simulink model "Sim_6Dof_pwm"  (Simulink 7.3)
settings: Solver=ode4  StartTime=0.0  StopTime=80  FixedStep=0.0005  MaxStep=0.0005  RelTol=1e-3
StopFcn:
  | Pl
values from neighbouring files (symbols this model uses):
  calfa = cos(alfa0*d2r)    [run.m]
  d2r = pi/180    (= 0.0174532925199)    [run.m]
  klr = [0.82083770557  -0.70145835124   0.75722294555   0.32691190448   0.14993771995;        0.55253708187   0.66141640307  -0.4963339086    0.20601876795  -0.07844376733]    [run.m]
  kls = [0.23009875115  -1.3857134134    0.5565800989    0.03843893525  0.1360972015;        0.22658853965   0.3268097242   -0.0904376422    0.0272194403  -0.00768778705]    [run.m]
  r2d = 180/pi    (= 57.2957795131)    [Pl.m]    (also in run.m)
  salfa = sin(alfa0*d2r)    [run.m]
  Thet0 = 43    [run.m]
  V0 = 18640    [run.m]
undefined symbols (not defined in the file or in its folder): A6d, B6d, C6d, D6d, KSmix, Pos_Thrust3

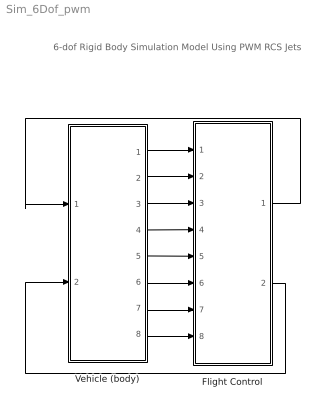
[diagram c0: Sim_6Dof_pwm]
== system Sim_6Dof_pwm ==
  note: 6-dof Rigid Body Simulation Model Using PWM RCS Jets
  Flight Control : Subsystem
  Vehicle (body) : Subsystem
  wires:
  Vehicle (body)/2(p) -> Flight Control/2(pb)
  Vehicle (body)/3(r) -> Flight Control/3(rb)
  Vehicle (body)/6(q) -> Flight Control/6(q)
  Vehicle (body)/5(thet) -> Flight Control/5(thet)
  Vehicle (body)/7(alf) -> Flight Control/7(alfa)
  Vehicle (body)/4(bet) -> Flight Control/4(beta)
  Vehicle (body)/1(phi) -> Flight Control/1(phi)
  Flight Control/2(Aer_pqr) -> Vehicle (body)/2(Aer_pqr)
  Vehicle (body)/8(Nz) -> Flight Control/8(Nz)
  Flight Control/1(Jet_pqr) -> Vehicle (body)/1(Jet_pqr_Nz)

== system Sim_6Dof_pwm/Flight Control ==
  note: Flight Control System
  phi : Inport  OutDataType=sfix(16)  OutScaling=2^0
  pb : Inport  Port=2  OutDataType=sfix(16)  OutScaling=2^0
  rb : Inport  Port=3  OutDataType=sfix(16)  OutScaling=2^0
  beta : Inport  Port=4  OutDataType=sfix(16)  OutScaling=2^0
  thet : Inport  Port=5  OutDataType=sfix(16)  OutScaling=2^0
  q : Inport  Port=6  OutDataType=sfix(16)  OutScaling=2^0
  alfa : Inport  Port=7  OutDataType=sfix(16)  OutScaling=2^0
  Nz : Inport  Port=8  OutDataType=sfix(16)  OutScaling=2^0
  2 deg  Alfa-Comd : Constant  Value=1*d2r  OutDataType=sfix(16)  OutScaling=2^0
  30 deg  phi-cmd : Constant  Value=40*d2r  OutDataType=sfix(16)  OutScaling=2^0
  Body 2 Stabil : Subsystem
  Lateral  Flight Control : Subsystem
  Mix : Subsystem
  Mux1 : Mux  Inputs=[3,1]
  Pitch Flight Control : Subsystem
  Jet_pqr : Outport  OutDataType=sfix(16)  OutScaling=2^0
  Aer_pqr : Outport  Port=2  OutDataType=sfix(16)  OutScaling=2^0
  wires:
  Lateral  Flight Control/1(rcs_PR) -> Mix/1(Rcs_PR)
  Lateral  Flight Control/2(aero_PR) -> Mix/2(Aer_PR)
  Pitch Flight Control/1(rcs_Q) -> Mix/3(Rcs_Q)
  Pitch Flight Control/2(aero_Q) -> Mix/4(Aer_Q)
  beta/1 -> Lateral  Flight Control/3(beta)
  Mix/2(Aer_pqr) -> Aer_pqr/1  "3"
  thet/1 -> Pitch Flight Control/1(thet)
  q/1 -> Pitch Flight Control/2(q)
  alfa/1 -> Pitch Flight Control/3(alf)
  Body 2 Stabil/2(r_s) -> Lateral  Flight Control/2(rs)
  Body 2 Stabil/1(p_s) -> Lateral  Flight Control/1(ps)
  rb/1 -> Body 2 Stabil/3(r_b)
  pb/1 -> Body 2 Stabil/2(p_b)
  phi/1 -> Body 2 Stabil/1(phi)
  Nz/1 -> Pitch Flight Control/4(Nz)
  Mix/1(Jet_pqr) -> Mux1/1  "3"
  2 deg  Alfa-Comd/1 -> Pitch Flight Control/5(alf-cmd)
  30 deg  phi-cmd/1 -> Lateral  Flight Control/4(phi-cmd)
  Pitch Flight Control/3(Nzfb) -> Mux1/2
  Mux1/1 -> Jet_pqr/1

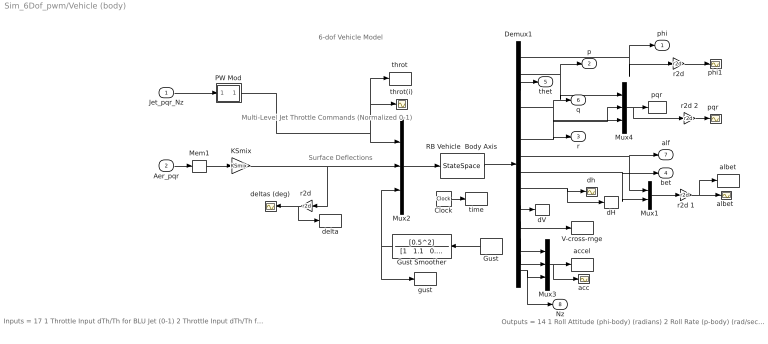
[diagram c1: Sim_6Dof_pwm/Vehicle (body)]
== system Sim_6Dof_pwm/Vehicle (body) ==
  note: Surface Deflections
  note: Multi-Level Jet Throttle Commands (Normalized 0-1)
  note: 6-dof Vehicle Model
  note: Inputs = 17 1 Throttle Input dTh/Th for BLU Jet (0-1) 2 Throttle Input dTh/Th for BRU Jet (0-1) 3 Throttle Input dTh/Th for BLD Jet (0-1) 4 Throttle Input dTh/Th for BRD Jet (0-1) 5 Throttle Input dTh/Th for BL+Y Jet (0-1) 6 Throttle Input dTh/Th for BR-Y Jet (0-1) 7 Throttle Input dTh/Th for FU Jet (0-1) 8 Throttle Input dTh/Th for FLD Jet (0-1) 9 Throttle Input dTh/Th for FRD Jet (0-1) 10 Throttle Input dTh/Th for FL+Y Jet (0-1) 11 Throttle Input dTh/Th for FR-Y Jet (0-1) 12 Left Outbrd Elevon Deflection (radians) 13 Left Inboard Elevon Deflection (radians) 14 Right Inbrd Elevon Deflection (radians) 15 Right Outbrd Elevon Deflection (radians) 16 Vertical Rudder Deflection (radians) 17 Gust Veloc, Azim-Elev Angles=(45,90) (deg)
  note: Outputs = 14 1 Roll Attitude (phi-body) (radians) 2 Roll Rate (p-body) (rad/sec) 3 Pitch Attitude (thet-bdy) (radians) 4 Pitch Rate (q-body) (rad/sec) 5 Yaw Attitude (psi-body) (radians) 6 Yaw Rate (r-body) (rad/sec) 7 Angle of attack, alfa, (radians) 8 Angle of sideslip, beta, (radian) 9 Change in Altitude, delta-h, (feet) 10 Forward Acceleration (V-dot) (ft/sec) 11 Cross Range Velocity (Vcr) (ft/sec) 12 CG Acceleration along X axis, (ft/sec^2) 13 CG Acceleration along Y axis, (ft/sec^2) 14 CG Acceleration along Z axis, (ft/sec^2)
  Jet_pqr_Nz : Inport  OutDataType=sfix(16)  OutScaling=2^0
  Aer_pqr : Inport  Port=2  OutDataType=sfix(16)  OutScaling=2^0
  Clock : Clock
  Demux1 : Demux  Outputs=14
  Gust : DiscretePulseGenerator  PulseType=Time based  Amplitude=50  Period=500  PulseWidth=10  PhaseDelay=0  SampleTime=1
  Gust Smoother : TransferFcn  Numerator=[0.5^2]  Denominator="[1   1.1   0.5^2]"
  KSmix : Gain  Gain=KSmix  Multiplication=Matrix(K*u)  ParameterDataType=sfix(16)  ParameterScaling=2^0  OutDataType=sfix(16)  OutScaling=2^0
  Mem1 : Memory
  Mux1 : Mux  Inputs=2
  Mux2 : Mux  Inputs=[11, 5, 1]
  Mux3 : Mux  Inputs=3
  Mux4 : Mux  Inputs=3
  PW Mod : Subsystem
  RB Vehicle  Body Axis : StateSpace  A=A6d  B=B6d  C=C6d  D=D6d
  V-cross-rnge : ToWorkspace  VariableName=Vxrng  SampleTime=-1  SaveFormat=Array
  acc : Scope
  accel : ToWorkspace  VariableName=accel  SampleTime=-1  SaveFormat=Array
  albet : ToWorkspace  VariableName=albet  SampleTime=-1  SaveFormat=Array
  "albet " : Scope
  dH : ToWorkspace  VariableName=dH  SampleTime=-1  SaveFormat=Array
  dV : ToWorkspace  VariableName=dV  SampleTime=-1  SaveFormat=Array
  delta : ToWorkspace  VariableName=delta  SampleTime=-1  SaveFormat=Array
  deltas (deg) : Scope
  dh : Scope
  gust : ToWorkspace  VariableName=gust  SampleTime=-1  SaveFormat=Array
  phi1 : Scope
  pqr : ToWorkspace  VariableName=pqr  SampleTime=-1  SaveFormat=Array
  "pqr  " : Scope
  r2d : Gain  Gain=r2d  ParameterDataType=sfix(16)  ParameterScaling=2^0  OutDataType=sfix(16)  OutScaling=2^0
  "r2d " : Gain  Gain=r2d  ParameterDataType=sfix(16)  ParameterScaling=2^0  OutDataType=sfix(16)  OutScaling=2^0
  r2d 1 : Gain  Gain=r2d  ParameterDataType=sfix(16)  ParameterScaling=2^0  OutDataType=sfix(16)  OutScaling=2^0
  r2d 2 : Gain  Gain=r2d  ParameterDataType=sfix(16)  ParameterScaling=2^0  OutDataType=sfix(16)  OutScaling=2^0
  throt : ToWorkspace  VariableName=throt  SampleTime=-1  SaveFormat=Array
  throt(i) : Scope
  time : ToWorkspace  VariableName=time  SampleTime=-1  SaveFormat=Array
  phi : Outport  OutDataType=sfix(16)  OutScaling=2^0
  p : Outport  Port=2  OutDataType=sfix(16)  OutScaling=2^0
  r : Outport  Port=3  OutDataType=sfix(16)  OutScaling=2^0
  bet : Outport  Port=4  OutDataType=sfix(16)  OutScaling=2^0
  thet : Outport  Port=5  OutDataType=sfix(16)  OutScaling=2^0
  q : Outport  Port=6  OutDataType=sfix(16)  OutScaling=2^0
  alf : Outport  Port=7  OutDataType=sfix(16)  OutScaling=2^0
  Nz : Outport  Port=8  OutDataType=sfix(16)  OutScaling=2^0
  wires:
  Mux2/1 -> RB Vehicle  Body Axis/1
  KSmix/1 -> Mux2/2, "r2d "/1
  Demux1/2 -> p/1, Mux4/1
  Demux1/4 -> q/1, Mux4/2
  Demux1/6 -> r/1, Mux4/3
  Demux1/7 -> alf/1, Mux1/1
  Demux1/8 -> bet/1, Mux1/2
  Aer_pqr/1 -> Mem1/1
  Demux1/3 -> thet/1
  "r2d "/1 -> deltas (deg)/1, delta/1
  Demux1/1 -> phi/1, r2d/1
  RB Vehicle  Body Axis/1 -> Demux1/1
  Demux1/9 -> dh/1, dH/1
  Demux1/10 -> dV/1
  r2d 1/1 -> "albet "/1, albet/1
  Demux1/11 -> V-cross-rnge/1
  Gust Smoother/1 -> gust/1, Mux2/3
  r2d/1 -> phi1/1
  Jet_pqr_Nz/1 -> PW Mod/1(In)
  Mem1/1 -> KSmix/1
  Clock/1 -> time/1
  Mux1/1 -> r2d 1/1
  Demux1/14 -> Mux3/3, Nz/1
  Demux1/13 -> Mux3/2
  Demux1/12 -> Mux3/1
  Mux3/1 -> accel/1, acc/1
  Mux4/1 -> pqr/1, r2d 2/1
  r2d 2/1 -> "pqr  "/1
  Gust/1 -> Gust Smoother/1
  PW Mod/1(Ot) -> Mux2/1, throt(i)/1, throt/1

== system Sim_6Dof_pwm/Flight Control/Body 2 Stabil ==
  note: Body to Stability Axes Transformation
  phi : Inport  OutDataType=sfix(16)  OutScaling=2^0
  p_b : Inport  Port=2  OutDataType=sfix(16)  OutScaling=2^0
  r_b : Inport  Port=3  OutDataType=sfix(16)  OutScaling=2^0
  Mux1 : Mux  Inputs=2
  Sum1 : Sum  Inputs=+|+  OutDataType=sfix(16)  OutScaling=2^0
  Sum2 : Sum  Inputs=+|-  OutDataType=sfix(16)  OutScaling=2^0
  Sum3 : Sum  Inputs=|++  OutDataType=sfix(16)  OutScaling=2^0
  Sum4 : Sum  Inputs=|+-  OutDataType=sfix(16)  OutScaling=2^0
  calfa : Gain  Gain=calfa  ParameterDataType=sfix(16)  ParameterScaling=2^0  OutDataType=sfix(16)  OutScaling=2^0
  "calfa " : Gain  Gain=calfa  ParameterDataType=sfix(16)  ParameterScaling=2^0  OutDataType=sfix(16)  OutScaling=2^0
  g cos(Thet0) /V0 : Gain  Gain=32.2*cos(Thet0*d2r)/V0  ParameterDataType=sfix(16)  ParameterScaling=2^0  OutDataType=sfix(16)  OutScaling=2^0
  g sin(Thet0) /V0 : Gain  Gain=32.2*sin(Thet0*d2r)/V0  ParameterDataType=sfix(16)  ParameterScaling=2^0  OutDataType=sfix(16)  OutScaling=2^0
  pr_stabil : ToWorkspace  VariableName=pr_st  SampleTime=-1  SaveFormat=Array
  salfa : Gain  Gain=salfa  ParameterDataType=sfix(16)  ParameterScaling=2^0  OutDataType=sfix(16)  OutScaling=2^0
  "salfa " : Gain  Gain=salfa  ParameterDataType=sfix(16)  ParameterScaling=2^0  OutDataType=sfix(16)  OutScaling=2^0
  p_s : Outport  OutDataType=sfix(16)  OutScaling=2^0
  r_s : Outport  Port=2  OutDataType=sfix(16)  OutScaling=2^0
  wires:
  Sum1/1 -> p_s/1, Mux1/1
  Sum2/1 -> r_s/1, Mux1/2
  p_b/1 -> Sum3/1
  r_b/1 -> Sum4/1
  g cos(Thet0) /V0/1 -> Sum3/2
  g sin(Thet0) /V0/1 -> Sum4/2
  phi/1 -> g cos(Thet0) /V0/1, g sin(Thet0) /V0/1
  Sum4/1 -> "calfa "/1, salfa/1
  Sum3/1 -> "salfa "/1, calfa/1
  calfa/1 -> Sum1/1
  salfa/1 -> Sum1/2
  "calfa "/1 -> Sum2/1
  "salfa "/1 -> Sum2/2
  Mux1/1 -> pr_stabil/1

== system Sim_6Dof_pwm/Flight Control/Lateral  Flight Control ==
  note: Lateral Flight Control System
  ps : Inport  OutDataType=sfix(16)  OutScaling=2^0
  rs : Inport  Port=2  OutDataType=sfix(16)  OutScaling=2^0
  beta : Inport  Port=3  OutDataType=sfix(16)  OutScaling=2^0
  phi-cmd : Inport  Port=4  OutDataType=sfix(16)  OutScaling=2^0
  5 state Aero feedback : Gain  Gain=-kls  Multiplication=Matrix(K*u)  ParameterDataType=sfix(16)  ParameterScaling=2^0  OutDataType=sfix(16)  OutScaling=2^0
  5 state RCS feedback : Gain  Gain=-klr  Multiplication=Matrix(K*u)  ParameterDataType=sfix(16)  ParameterScaling=2^0  OutDataType=sfix(16)  OutScaling=2^0
  Int : Integrator
  "Int " : Integrator
  Mux3 : Mux  Inputs=5
  Sum : Sum  Inputs=|+-  OutDataType=sfix(16)  OutScaling=2^0
  phi : Scope
  phi-cmd (rad) : ToWorkspace  VariableName=phi_cmd  SampleTime=-1  SaveFormat=Array
  phi-stabil : ToWorkspace  VariableName=phi_st  SampleTime=-1  SaveFormat=Array
  r2d : Gain  Gain=r2d  ParameterDataType=sfix(16)  ParameterScaling=2^0  OutDataType=sfix(16)  OutScaling=2^0
  rcs_PR : Outport  OutDataType=sfix(16)  OutScaling=2^0
  aero_PR : Outport  Port=2  OutDataType=sfix(16)  OutScaling=2^0
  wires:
  "Int "/1 -> Sum/1, r2d/1  "pint"
  Sum/1 -> Mux3/4
  Int/1 -> Mux3/5  "beti"
  beta/1 -> Int/1, Mux3/3
  ps/1 -> "Int "/1, Mux3/1
  Mux3/1 -> 5 state Aero feedback/1, 5 state RCS feedback/1
  rs/1 -> Mux3/2
  5 state RCS feedback/1 -> rcs_PR/1  "rcs(P,R)"
  5 state Aero feedback/1 -> aero_PR/1  "aero(P,R)"
  phi-cmd/1 -> Sum/2, phi-cmd (rad)/1
  r2d/1 -> phi/1, phi-stabil/1

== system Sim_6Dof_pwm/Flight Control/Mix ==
  Rcs_PR : Inport  OutDataType=sfix(16)  OutScaling=2^0
  Aer_PR : Inport  Port=2  OutDataType=sfix(16)  OutScaling=2^0
  Rcs_Q : Inport  Port=3  OutDataType=sfix(16)  OutScaling=2^0
  Aer_Q : Inport  Port=4  OutDataType=sfix(16)  OutScaling=2^0
  Demux1 : Demux  Outputs=2
  Demux2 : Demux  Outputs=2
  Mux1 : Mux  Inputs=3
  Mux2 : Mux  Inputs=3
  Jet_pqr : Outport  OutDataType=sfix(16)  OutScaling=2^0
  Aer_pqr : Outport  Port=2  OutDataType=sfix(16)  OutScaling=2^0
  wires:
  Demux1/1 -> Mux1/1
  Demux1/2 -> Mux1/3
  Demux2/1 -> Mux2/1
  Demux2/2 -> Mux2/3
  Mux1/1 -> Jet_pqr/1
  Rcs_PR/1 -> Demux1/1
  Aer_PR/1 -> Demux2/1
  Aer_Q/1 -> Mux2/2
  Mux2/1 -> Aer_pqr/1
  Rcs_Q/1 -> Mux1/2

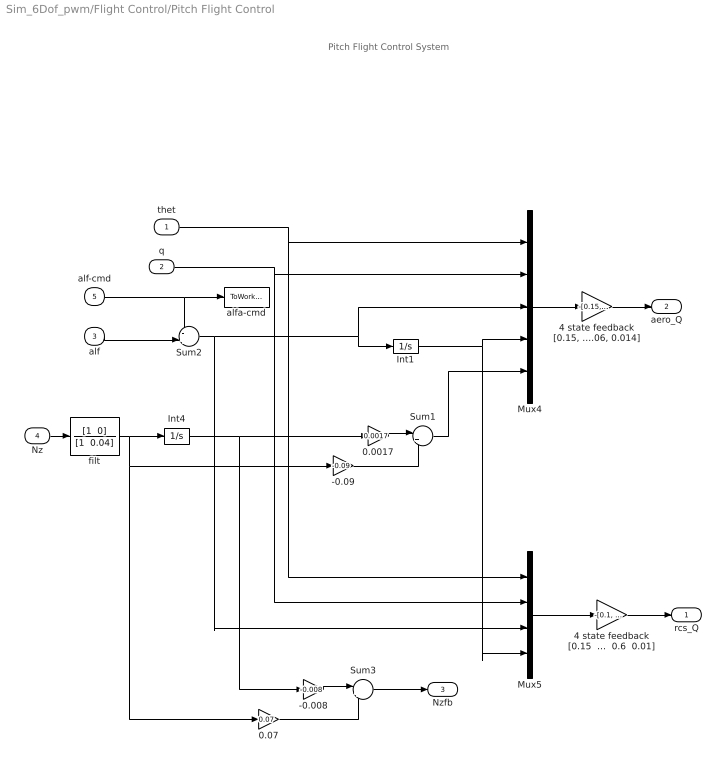
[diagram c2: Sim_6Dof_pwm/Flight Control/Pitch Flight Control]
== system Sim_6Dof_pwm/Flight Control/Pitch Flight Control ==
  note: Pitch Flight Control System
  thet : Inport  OutDataType=sfix(16)  OutScaling=2^0
  q : Inport  Port=2  OutDataType=sfix(16)  OutScaling=2^0
  alf : Inport  Port=3  OutDataType=sfix(16)  OutScaling=2^0
  Nz : Inport  Port=4  OutDataType=sfix(16)  OutScaling=2^0
  alf-cmd : Inport  Port=5  OutDataType=sfix(16)  OutScaling=2^0
  -0.008 : Gain  Gain=-0.008  ParameterDataType=sfix(16)  ParameterScaling=2^0  OutDataType=sfix(16)  OutScaling=2^0
  -0.09 : Gain  Gain=-0.09  ParameterDataType=sfix(16)  ParameterScaling=2^0  OutDataType=sfix(16)  OutScaling=2^0
  0.0017 : Gain  Gain=0.0017  ParameterDataType=sfix(16)  ParameterScaling=2^0  OutDataType=sfix(16)  OutScaling=2^0
  0.07 : Gain  Gain=0.07  ParameterDataType=sfix(16)  ParameterScaling=2^0  OutDataType=sfix(16)  OutScaling=2^0
  4 state feedback [0.15  1.8  0.6  0.01] : Gain  Gain="-[0.1,   1.8,   0.9,    0.01]"  Multiplication=Matrix(K*u)  ParameterDataType=sfix(16)  ParameterScaling=2^0  OutDataType=sfix(16)  OutScaling=2^0
  "4 state feedback [0.15, 2, 0.9, 0.06, 0.014]" : Gain  Gain="-[0.15,   2,   1.2,    0.09,   0.015]"  Multiplication=Matrix(K*u)  ParameterDataType=sfix(16)  ParameterScaling=2^0  OutDataType=sfix(16)  OutScaling=2^0
  Int1 : Integrator
  Int4 : Integrator
  Mux4 : Mux  Inputs=5
  Mux5 : Mux
  Sum1 : Sum  Inputs=|++  OutDataType=sfix(16)  OutScaling=2^0
  Sum2 : Sum  Inputs=-+|  OutDataType=sfix(16)  OutScaling=2^0
  Sum3 : Sum  Inputs=|++  OutDataType=sfix(16)  OutScaling=2^0
  alfa-cmd : ToWorkspace  VariableName=alfa_cmd  SampleTime=-1  SaveFormat=Array
  filt : TransferFcn  Numerator="[1  0]"  Denominator="[1  0.04]"
  rcs_Q : Outport  OutDataType=sfix(16)  OutScaling=2^0
  aero_Q : Outport  Port=2  OutDataType=sfix(16)  OutScaling=2^0
  Nzfb : Outport  Port=3  OutDataType=sfix(16)  OutScaling=2^0
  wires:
  alf-cmd/1 -> Sum2/1, alfa-cmd/1
  alf/1 -> Sum2/2
  filt/1 -> 0.07/1, -0.09/1, Int4/1
  Int4/1 -> -0.008/1, 0.0017/1
  -0.008/1 -> Sum3/1
  0.07/1 -> Sum3/2
  4 state feedback [0.15  1.8  0.6  0.01]/1 -> rcs_Q/1
  Mux5/1 -> 4 state feedback [0.15  1.8  0.6  0.01]/1
  "4 state feedback [0.15, 2, 0.9, 0.06, 0.014]"/1 -> aero_Q/1
  Mux4/1 -> "4 state feedback [0.15, 2, 0.9, 0.06, 0.014]"/1
  Sum1/1 -> Mux4/5
  Nz/1 -> filt/1
  -0.09/1 -> Sum1/2
  0.0017/1 -> Sum1/1
  q/1 -> Mux5/2, Mux4/2
  thet/1 -> Mux5/1, Mux4/1
  Sum2/1 -> Mux5/3, Mux4/3, Int1/1
  Int1/1 -> Mux5/4, Mux4/4
  Sum3/1 -> Nzfb/1

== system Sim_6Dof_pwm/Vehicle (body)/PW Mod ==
  note: Jet Selection Logic
  In : Inport  OutDataType=sfix(16)  OutScaling=2^0
  Demux2 : Demux  Outputs="[3  3  3  3  3  3  2  2  2  2  2  1]"
  Mem : Memory
  Mix Logic +ve thrusts : MATLABFcn  MATLABFcn=Pos_Thrust3(u(1:4) )  OutputDimensions=6*3 + 5*2 + 1  OutputSignalType=real
  Mux1 : Mux  Inputs=11
  PW Modulators : Subsystem
  error : Scope
  error-magn : ToWorkspace  VariableName=erm  SampleTime=-1  SaveFormat=Array
  Ot : Outport  OutDataType=sfix(16)  OutScaling=2^0
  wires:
  In/1 -> Mem/1
  Mux1/1 -> Ot/1
  Mem/1 -> Mix Logic +ve thrusts/1
  Demux2/1 -> PW Modulators/1(In)
  Demux2/2 -> PW Modulators/2(In1)
  Demux2/3 -> PW Modulators/3(In2)
  Demux2/4 -> PW Modulators/4(In3)
  Demux2/5 -> PW Modulators/5(In4)
  Demux2/6 -> PW Modulators/6(In5)
  Demux2/7 -> PW Modulators/7(In6)
  Demux2/8 -> PW Modulators/8(In7)
  Demux2/9 -> PW Modulators/9(In8)
  Demux2/10 -> PW Modulators/10(In9)
  Demux2/11 -> PW Modulators/11(In10)
  PW Modulators/1(O) -> Mux1/1
  PW Modulators/2(O1) -> Mux1/2
  PW Modulators/3(O2) -> Mux1/3
  PW Modulators/4(O3) -> Mux1/4
  PW Modulators/5(O4) -> Mux1/5
  PW Modulators/6(O5) -> Mux1/6
  PW Modulators/7(O6) -> Mux1/7
  PW Modulators/8(O7) -> Mux1/8
  PW Modulators/9(O8) -> Mux1/9
  PW Modulators/10(O9) -> Mux1/10
  PW Modulators/11(O10) -> Mux1/11
  Mix Logic +ve thrusts/1 -> Demux2/1
  Demux2/12 -> error/1, error-magn/1

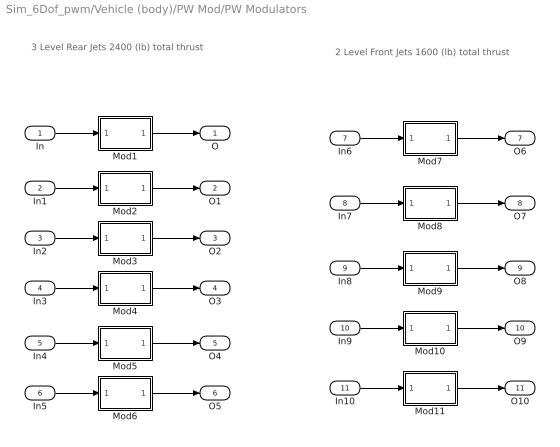
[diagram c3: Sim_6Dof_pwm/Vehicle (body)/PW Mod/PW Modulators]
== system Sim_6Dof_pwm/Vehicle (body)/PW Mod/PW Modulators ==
  note: 3 Level Rear Jets 2400 (lb) total thrust
  note: 2 Level Front Jets 1600 (lb) total thrust
  In : Inport  OutDataType=sfix(16)  OutScaling=2^0
  In1 : Inport  Port=2  OutDataType=sfix(16)  OutScaling=2^0
  In2 : Inport  Port=3  OutDataType=sfix(16)  OutScaling=2^0
  In3 : Inport  Port=4  OutDataType=sfix(16)  OutScaling=2^0
  In4 : Inport  Port=5  OutDataType=sfix(16)  OutScaling=2^0
  In5 : Inport  Port=6  OutDataType=sfix(16)  OutScaling=2^0
  In6 : Inport  Port=7  OutDataType=sfix(16)  OutScaling=2^0
  In7 : Inport  Port=8  OutDataType=sfix(16)  OutScaling=2^0
  In8 : Inport  Port=9  OutDataType=sfix(16)  OutScaling=2^0
  In9 : Inport  Port=10  OutDataType=sfix(16)  OutScaling=2^0
  In10 : Inport  Port=11  OutDataType=sfix(16)  OutScaling=2^0
  Mod1 : Subsystem
  Mod10 : Subsystem
  Mod11 : Subsystem
  Mod2 : Subsystem
  Mod3 : Subsystem
  Mod4 : Subsystem
  Mod5 : Subsystem
  Mod6 : Subsystem
  Mod7 : Subsystem
  Mod8 : Subsystem
  Mod9 : Subsystem
  O : Outport  OutDataType=sfix(16)  OutScaling=2^0
  O1 : Outport  Port=2  OutDataType=sfix(16)  OutScaling=2^0
  O2 : Outport  Port=3  OutDataType=sfix(16)  OutScaling=2^0
  O3 : Outport  Port=4  OutDataType=sfix(16)  OutScaling=2^0
  O4 : Outport  Port=5  OutDataType=sfix(16)  OutScaling=2^0
  O5 : Outport  Port=6  OutDataType=sfix(16)  OutScaling=2^0
  O6 : Outport  Port=7  OutDataType=sfix(16)  OutScaling=2^0
  O7 : Outport  Port=8  OutDataType=sfix(16)  OutScaling=2^0
  O8 : Outport  Port=9  OutDataType=sfix(16)  OutScaling=2^0
  O9 : Outport  Port=10  OutDataType=sfix(16)  OutScaling=2^0
  O10 : Outport  Port=11  OutDataType=sfix(16)  OutScaling=2^0
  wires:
  Mod1/1(O1) -> O/1
  In/1 -> Mod1/1(In1)
  Mod2/1(O1) -> O1/1
  In1/1 -> Mod2/1(In1)
  Mod3/1(O1) -> O2/1
  In2/1 -> Mod3/1(In1)
  Mod4/1(O1) -> O3/1
  In3/1 -> Mod4/1(In1)
  Mod5/1(O1) -> O4/1
  In4/1 -> Mod5/1(In1)
  Mod6/1(O1) -> O5/1
  In5/1 -> Mod6/1(In1)
  Mod7/1(O1) -> O6/1
  In6/1 -> Mod7/1(In1)
  Mod8/1(O1) -> O7/1
  In7/1 -> Mod8/1(In1)
  Mod9/1(O1) -> O8/1
  In8/1 -> Mod9/1(In1)
  Mod10/1(O1) -> O9/1
  In9/1 -> Mod10/1(In1)
  Mod11/1(O1) -> O10/1
  In10/1 -> Mod11/1(In1)

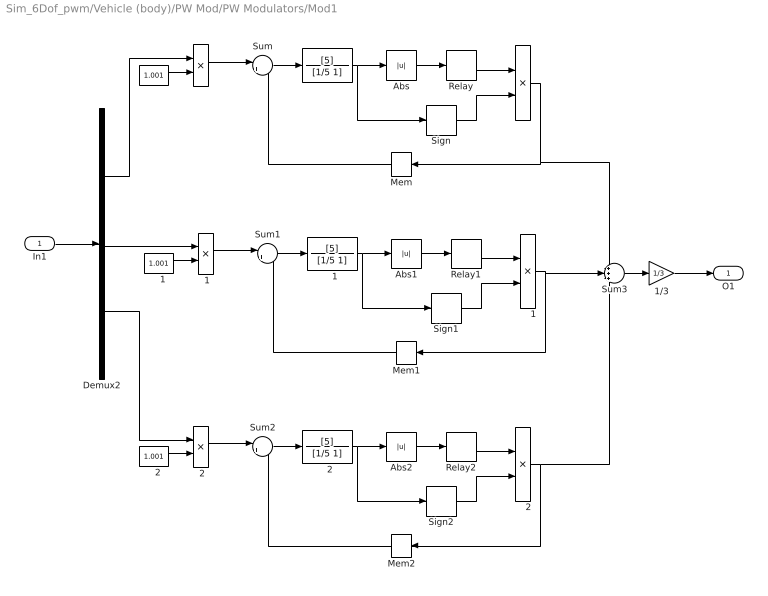
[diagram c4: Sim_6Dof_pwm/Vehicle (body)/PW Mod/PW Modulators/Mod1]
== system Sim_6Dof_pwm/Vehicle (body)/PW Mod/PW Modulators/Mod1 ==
  In1 : Inport  OutDataType=sfix(16)  OutScaling=2^0
  " " : Product  OutDataType=sfix(16)  OutScaling=2^0
  "  " : TransferFcn  Numerator=[5]  Denominator=[1/5 1]
  "   " : Constant  Value=1.001  OutDataType=sfix(16)  OutScaling=2^0
  "    " : Product  OutDataType=sfix(16)  OutScaling=2^0
  "    1" : Product  OutDataType=sfix(16)  OutScaling=2^0
  "    2" : Product  OutDataType=sfix(16)  OutScaling=2^0
  "   1" : Constant  Value=1.001  OutDataType=sfix(16)  OutScaling=2^0
  "   2" : Constant  Value=1.001  OutDataType=sfix(16)  OutScaling=2^0
  "  1" : TransferFcn  Numerator=[5]  Denominator=[1/5 1]
  "  2" : TransferFcn  Numerator=[5]  Denominator=[1/5 1]
  " 1" : Product  OutDataType=sfix(16)  OutScaling=2^0
  " 2" : Product  OutDataType=sfix(16)  OutScaling=2^0
  1/3 : Gain  Gain=1/3  ParameterDataType=sfix(16)  ParameterScaling=2^0  OutDataType=sfix(16)  OutScaling=2^0
  Abs : Abs
  Abs1 : Abs
  Abs2 : Abs
  Demux2 : Demux  Outputs=3
  Mem : Memory
  Mem1 : Memory
  Mem2 : Memory
  Relay : Relay  OnSwitchValue=0.5  OffSwitchValue=0.5  OutDataType=sfix(16)  OutScaling=2^0
  Relay1 : Relay  OnSwitchValue=0.5  OffSwitchValue=0.5  OutDataType=sfix(16)  OutScaling=2^0
  Relay2 : Relay  OnSwitchValue=0.5  OffSwitchValue=0.5  OutDataType=sfix(16)  OutScaling=2^0
  Sign : Signum
  Sign1 : Signum
  Sign2 : Signum
  Sum : Sum  Inputs=|+-  OutDataType=sfix(16)  OutScaling=2^0
  Sum1 : Sum  Inputs=|+-  OutDataType=sfix(16)  OutScaling=2^0
  Sum2 : Sum  Inputs=|+-  OutDataType=sfix(16)  OutScaling=2^0
  Sum3 : Sum  Inputs=+++  OutDataType=sfix(16)  OutScaling=2^0
  O1 : Outport  OutDataType=sfix(16)  OutScaling=2^0
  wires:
  "    "/1 -> Mem/1, Sum3/1
  Mem/1 -> Sum/2
  Sign/1 -> "    "/2
  Relay/1 -> "    "/1
  Abs/1 -> Relay/1
  "  "/1 -> Sign/1, Abs/1
  Sum/1 -> "  "/1
  "   "/1 -> " "/2
  " "/1 -> Sum/1
  "    1"/1 -> Mem1/1, Sum3/2
  Mem1/1 -> Sum1/2
  Sign1/1 -> "    1"/2
  Relay1/1 -> "    1"/1
  Abs1/1 -> Relay1/1
  "  1"/1 -> Sign1/1, Abs1/1
  Sum1/1 -> "  1"/1
  "   1"/1 -> " 1"/2
  " 1"/1 -> Sum1/1
  "    2"/1 -> Mem2/1, Sum3/3
  Mem2/1 -> Sum2/2
  Sign2/1 -> "    2"/2
  Relay2/1 -> "    2"/1
  Abs2/1 -> Relay2/1
  "  2"/1 -> Sign2/1, Abs2/1
  Sum2/1 -> "  2"/1
  "   2"/1 -> " 2"/2
  " 2"/1 -> Sum2/1
  Demux2/2 -> " 1"/1
  Demux2/1 -> " "/1
  Demux2/3 -> " 2"/1
  In1/1 -> Demux2/1
  Sum3/1 -> 1/3/1
  1/3/1 -> O1/1

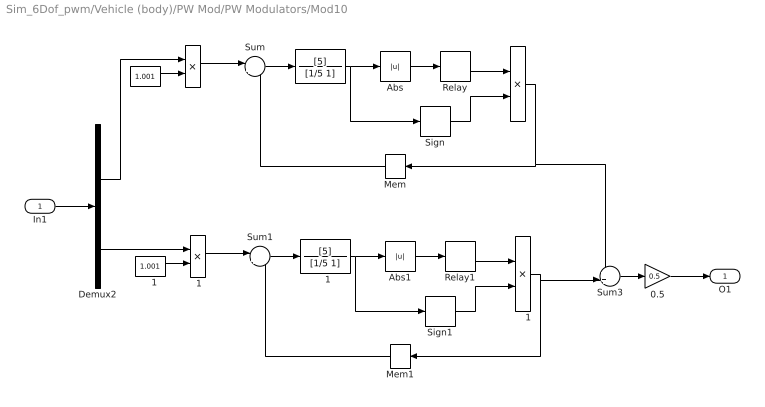
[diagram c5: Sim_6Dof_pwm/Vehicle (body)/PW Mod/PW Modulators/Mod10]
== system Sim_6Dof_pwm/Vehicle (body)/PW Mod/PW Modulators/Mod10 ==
  In1 : Inport  OutDataType=sfix(16)  OutScaling=2^0
  " " : Product  OutDataType=sfix(16)  OutScaling=2^0
  "  " : TransferFcn  Numerator=[5]  Denominator=[1/5 1]
  "   " : Constant  Value=1.001  OutDataType=sfix(16)  OutScaling=2^0
  "    " : Product  OutDataType=sfix(16)  OutScaling=2^0
  "    1" : Product  OutDataType=sfix(16)  OutScaling=2^0
  "   1" : Constant  Value=1.001  OutDataType=sfix(16)  OutScaling=2^0
  "  1" : TransferFcn  Numerator=[5]  Denominator=[1/5 1]
  " 1" : Product  OutDataType=sfix(16)  OutScaling=2^0
  0.5 : Gain  Gain=0.5  ParameterDataType=sfix(16)  ParameterScaling=2^0  OutDataType=sfix(16)  OutScaling=2^0
  Abs : Abs
  Abs1 : Abs
  Demux2 : Demux  Outputs=2
  Mem : Memory
  Mem1 : Memory
  Relay : Relay  OnSwitchValue=0.5  OffSwitchValue=0.5  OutDataType=sfix(16)  OutScaling=2^0
  Relay1 : Relay  OnSwitchValue=0.5  OffSwitchValue=0.5  OutDataType=sfix(16)  OutScaling=2^0
  Sign : Signum
  Sign1 : Signum
  Sum : Sum  Inputs=|+-  OutDataType=sfix(16)  OutScaling=2^0
  Sum1 : Sum  Inputs=|+-  OutDataType=sfix(16)  OutScaling=2^0
  Sum3 : Sum  Inputs=++|  OutDataType=sfix(16)  OutScaling=2^0
  O1 : Outport  OutDataType=sfix(16)  OutScaling=2^0
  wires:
  "    "/1 -> Mem/1, Sum3/1
  Mem/1 -> Sum/2
  Sign/1 -> "    "/2
  Relay/1 -> "    "/1
  Abs/1 -> Relay/1
  "  "/1 -> Sign/1, Abs/1
  Sum/1 -> "  "/1
  "   "/1 -> " "/2
  " "/1 -> Sum/1
  "    1"/1 -> Mem1/1, Sum3/2
  Mem1/1 -> Sum1/2
  Sign1/1 -> "    1"/2
  Relay1/1 -> "    1"/1
  Abs1/1 -> Relay1/1
  "  1"/1 -> Sign1/1, Abs1/1
  Sum1/1 -> "  1"/1
  "   1"/1 -> " 1"/2
  " 1"/1 -> Sum1/1
  Demux2/2 -> " 1"/1
  Demux2/1 -> " "/1
  In1/1 -> Demux2/1
  Sum3/1 -> 0.5/1
  0.5/1 -> O1/1

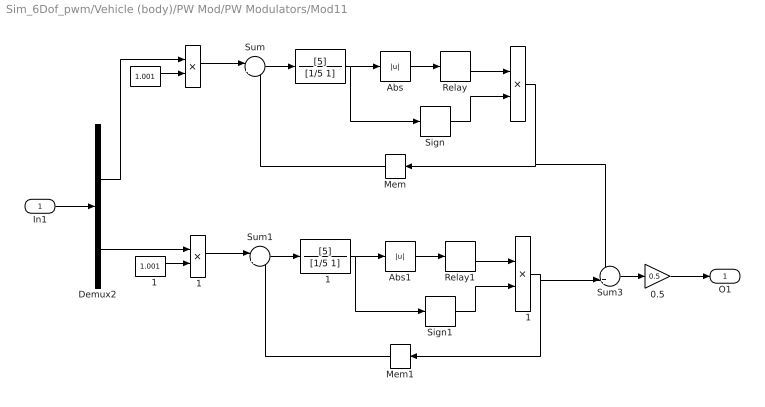
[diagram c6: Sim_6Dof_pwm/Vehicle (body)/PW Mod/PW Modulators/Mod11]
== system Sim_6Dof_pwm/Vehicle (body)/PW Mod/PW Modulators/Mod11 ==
  In1 : Inport  OutDataType=sfix(16)  OutScaling=2^0
  " " : Product  OutDataType=sfix(16)  OutScaling=2^0
  "  " : TransferFcn  Numerator=[5]  Denominator=[1/5 1]
  "   " : Constant  Value=1.001  OutDataType=sfix(16)  OutScaling=2^0
  "    " : Product  OutDataType=sfix(16)  OutScaling=2^0
  "    1" : Product  OutDataType=sfix(16)  OutScaling=2^0
  "   1" : Constant  Value=1.001  OutDataType=sfix(16)  OutScaling=2^0
  "  1" : TransferFcn  Numerator=[5]  Denominator=[1/5 1]
  " 1" : Product  OutDataType=sfix(16)  OutScaling=2^0
  0.5 : Gain  Gain=0.5  ParameterDataType=sfix(16)  ParameterScaling=2^0  OutDataType=sfix(16)  OutScaling=2^0
  Abs : Abs
  Abs1 : Abs
  Demux2 : Demux  Outputs=2
  Mem : Memory
  Mem1 : Memory
  Relay : Relay  OnSwitchValue=0.5  OffSwitchValue=0.5  OutDataType=sfix(16)  OutScaling=2^0
  Relay1 : Relay  OnSwitchValue=0.5  OffSwitchValue=0.5  OutDataType=sfix(16)  OutScaling=2^0
  Sign : Signum
  Sign1 : Signum
  Sum : Sum  Inputs=|+-  OutDataType=sfix(16)  OutScaling=2^0
  Sum1 : Sum  Inputs=|+-  OutDataType=sfix(16)  OutScaling=2^0
  Sum3 : Sum  Inputs=++|  OutDataType=sfix(16)  OutScaling=2^0
  O1 : Outport  OutDataType=sfix(16)  OutScaling=2^0
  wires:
  "    "/1 -> Mem/1, Sum3/1
  Mem/1 -> Sum/2
  Sign/1 -> "    "/2
  Relay/1 -> "    "/1
  Abs/1 -> Relay/1
  "  "/1 -> Sign/1, Abs/1
  Sum/1 -> "  "/1
  "   "/1 -> " "/2
  " "/1 -> Sum/1
  "    1"/1 -> Mem1/1, Sum3/2
  Mem1/1 -> Sum1/2
  Sign1/1 -> "    1"/2
  Relay1/1 -> "    1"/1
  Abs1/1 -> Relay1/1
  "  1"/1 -> Sign1/1, Abs1/1
  Sum1/1 -> "  1"/1
  "   1"/1 -> " 1"/2
  " 1"/1 -> Sum1/1
  Demux2/2 -> " 1"/1
  Demux2/1 -> " "/1
  In1/1 -> Demux2/1
  Sum3/1 -> 0.5/1
  0.5/1 -> O1/1

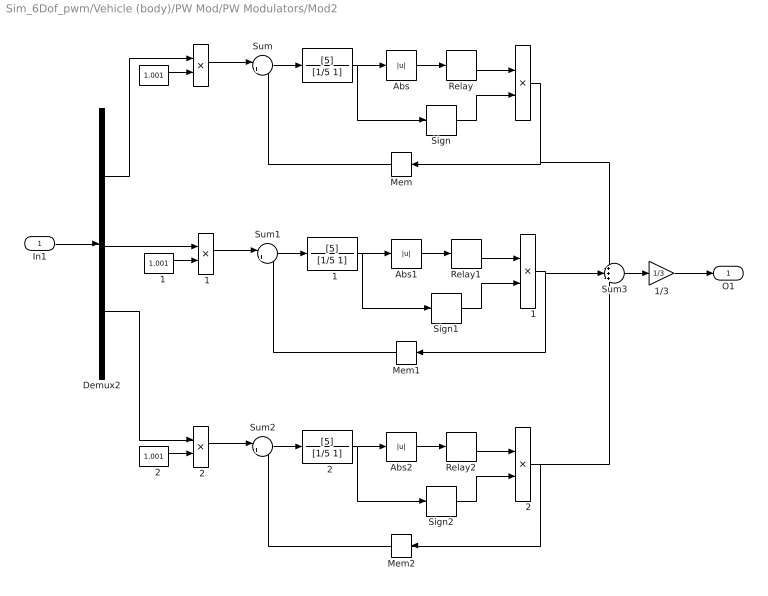
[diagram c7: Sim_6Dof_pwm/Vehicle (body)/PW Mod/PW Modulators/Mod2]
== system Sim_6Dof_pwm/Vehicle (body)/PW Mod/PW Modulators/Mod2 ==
  In1 : Inport  OutDataType=sfix(16)  OutScaling=2^0
  " " : Product  OutDataType=sfix(16)  OutScaling=2^0
  "  " : TransferFcn  Numerator=[5]  Denominator=[1/5 1]
  "   " : Constant  Value=1.001  OutDataType=sfix(16)  OutScaling=2^0
  "    " : Product  OutDataType=sfix(16)  OutScaling=2^0
  "    1" : Product  OutDataType=sfix(16)  OutScaling=2^0
  "    2" : Product  OutDataType=sfix(16)  OutScaling=2^0
  "   1" : Constant  Value=1.001  OutDataType=sfix(16)  OutScaling=2^0
  "   2" : Constant  Value=1.001  OutDataType=sfix(16)  OutScaling=2^0
  "  1" : TransferFcn  Numerator=[5]  Denominator=[1/5 1]
  "  2" : TransferFcn  Numerator=[5]  Denominator=[1/5 1]
  " 1" : Product  OutDataType=sfix(16)  OutScaling=2^0
  " 2" : Product  OutDataType=sfix(16)  OutScaling=2^0
  1/3 : Gain  Gain=1/3  ParameterDataType=sfix(16)  ParameterScaling=2^0  OutDataType=sfix(16)  OutScaling=2^0
  Abs : Abs
  Abs1 : Abs
  Abs2 : Abs
  Demux2 : Demux  Outputs=3
  Mem : Memory
  Mem1 : Memory
  Mem2 : Memory
  Relay : Relay  OnSwitchValue=0.5  OffSwitchValue=0.5  OutDataType=sfix(16)  OutScaling=2^0
  Relay1 : Relay  OnSwitchValue=0.5  OffSwitchValue=0.5  OutDataType=sfix(16)  OutScaling=2^0
  Relay2 : Relay  OnSwitchValue=0.5  OffSwitchValue=0.5  OutDataType=sfix(16)  OutScaling=2^0
  Sign : Signum
  Sign1 : Signum
  Sign2 : Signum
  Sum : Sum  Inputs=|+-  OutDataType=sfix(16)  OutScaling=2^0
  Sum1 : Sum  Inputs=|+-  OutDataType=sfix(16)  OutScaling=2^0
  Sum2 : Sum  Inputs=|+-  OutDataType=sfix(16)  OutScaling=2^0
  Sum3 : Sum  Inputs=+++  OutDataType=sfix(16)  OutScaling=2^0
  O1 : Outport  OutDataType=sfix(16)  OutScaling=2^0
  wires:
  "    "/1 -> Mem/1, Sum3/1
  Mem/1 -> Sum/2
  Sign/1 -> "    "/2
  Relay/1 -> "    "/1
  Abs/1 -> Relay/1
  "  "/1 -> Sign/1, Abs/1
  Sum/1 -> "  "/1
  "   "/1 -> " "/2
  " "/1 -> Sum/1
  "    1"/1 -> Mem1/1, Sum3/2
  Mem1/1 -> Sum1/2
  Sign1/1 -> "    1"/2
  Relay1/1 -> "    1"/1
  Abs1/1 -> Relay1/1
  "  1"/1 -> Sign1/1, Abs1/1
  Sum1/1 -> "  1"/1
  "   1"/1 -> " 1"/2
  " 1"/1 -> Sum1/1
  "    2"/1 -> Mem2/1, Sum3/3
  Mem2/1 -> Sum2/2
  Sign2/1 -> "    2"/2
  Relay2/1 -> "    2"/1
  Abs2/1 -> Relay2/1
  "  2"/1 -> Sign2/1, Abs2/1
  Sum2/1 -> "  2"/1
  "   2"/1 -> " 2"/2
  " 2"/1 -> Sum2/1
  Demux2/2 -> " 1"/1
  Demux2/1 -> " "/1
  Demux2/3 -> " 2"/1
  In1/1 -> Demux2/1
  Sum3/1 -> 1/3/1
  1/3/1 -> O1/1

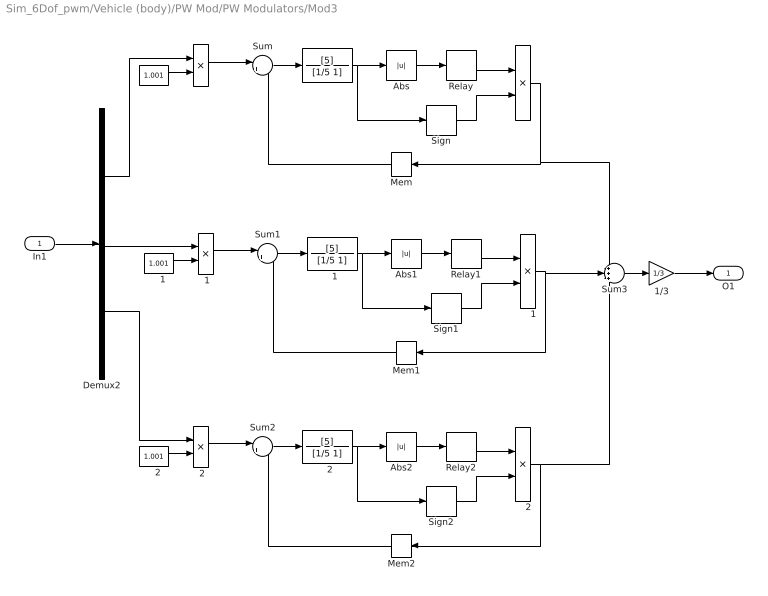
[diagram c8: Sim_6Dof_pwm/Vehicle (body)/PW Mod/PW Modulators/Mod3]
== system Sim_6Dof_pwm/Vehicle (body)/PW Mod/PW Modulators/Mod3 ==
  In1 : Inport  OutDataType=sfix(16)  OutScaling=2^0
  " " : Product  OutDataType=sfix(16)  OutScaling=2^0
  "  " : TransferFcn  Numerator=[5]  Denominator=[1/5 1]
  "   " : Constant  Value=1.001  OutDataType=sfix(16)  OutScaling=2^0
  "    " : Product  OutDataType=sfix(16)  OutScaling=2^0
  "    1" : Product  OutDataType=sfix(16)  OutScaling=2^0
  "    2" : Product  OutDataType=sfix(16)  OutScaling=2^0
  "   1" : Constant  Value=1.001  OutDataType=sfix(16)  OutScaling=2^0
  "   2" : Constant  Value=1.001  OutDataType=sfix(16)  OutScaling=2^0
  "  1" : TransferFcn  Numerator=[5]  Denominator=[1/5 1]
  "  2" : TransferFcn  Numerator=[5]  Denominator=[1/5 1]
  " 1" : Product  OutDataType=sfix(16)  OutScaling=2^0
  " 2" : Product  OutDataType=sfix(16)  OutScaling=2^0
  1/3 : Gain  Gain=1/3  ParameterDataType=sfix(16)  ParameterScaling=2^0  OutDataType=sfix(16)  OutScaling=2^0
  Abs : Abs
  Abs1 : Abs
  Abs2 : Abs
  Demux2 : Demux  Outputs=3
  Mem : Memory
  Mem1 : Memory
  Mem2 : Memory
  Relay : Relay  OnSwitchValue=0.5  OffSwitchValue=0.5  OutDataType=sfix(16)  OutScaling=2^0
  Relay1 : Relay  OnSwitchValue=0.5  OffSwitchValue=0.5  OutDataType=sfix(16)  OutScaling=2^0
  Relay2 : Relay  OnSwitchValue=0.5  OffSwitchValue=0.5  OutDataType=sfix(16)  OutScaling=2^0
  Sign : Signum
  Sign1 : Signum
  Sign2 : Signum
  Sum : Sum  Inputs=|+-  OutDataType=sfix(16)  OutScaling=2^0
  Sum1 : Sum  Inputs=|+-  OutDataType=sfix(16)  OutScaling=2^0
  Sum2 : Sum  Inputs=|+-  OutDataType=sfix(16)  OutScaling=2^0
  Sum3 : Sum  Inputs=+++  OutDataType=sfix(16)  OutScaling=2^0
  O1 : Outport  OutDataType=sfix(16)  OutScaling=2^0
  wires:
  "    "/1 -> Mem/1, Sum3/1
  Mem/1 -> Sum/2
  Sign/1 -> "    "/2
  Relay/1 -> "    "/1
  Abs/1 -> Relay/1
  "  "/1 -> Sign/1, Abs/1
  Sum/1 -> "  "/1
  "   "/1 -> " "/2
  " "/1 -> Sum/1
  "    1"/1 -> Mem1/1, Sum3/2
  Mem1/1 -> Sum1/2
  Sign1/1 -> "    1"/2
  Relay1/1 -> "    1"/1
  Abs1/1 -> Relay1/1
  "  1"/1 -> Sign1/1, Abs1/1
  Sum1/1 -> "  1"/1
  "   1"/1 -> " 1"/2
  " 1"/1 -> Sum1/1
  "    2"/1 -> Mem2/1, Sum3/3
  Mem2/1 -> Sum2/2
  Sign2/1 -> "    2"/2
  Relay2/1 -> "    2"/1
  Abs2/1 -> Relay2/1
  "  2"/1 -> Sign2/1, Abs2/1
  Sum2/1 -> "  2"/1
  "   2"/1 -> " 2"/2
  " 2"/1 -> Sum2/1
  Demux2/2 -> " 1"/1
  Demux2/1 -> " "/1
  Demux2/3 -> " 2"/1
  In1/1 -> Demux2/1
  Sum3/1 -> 1/3/1
  1/3/1 -> O1/1

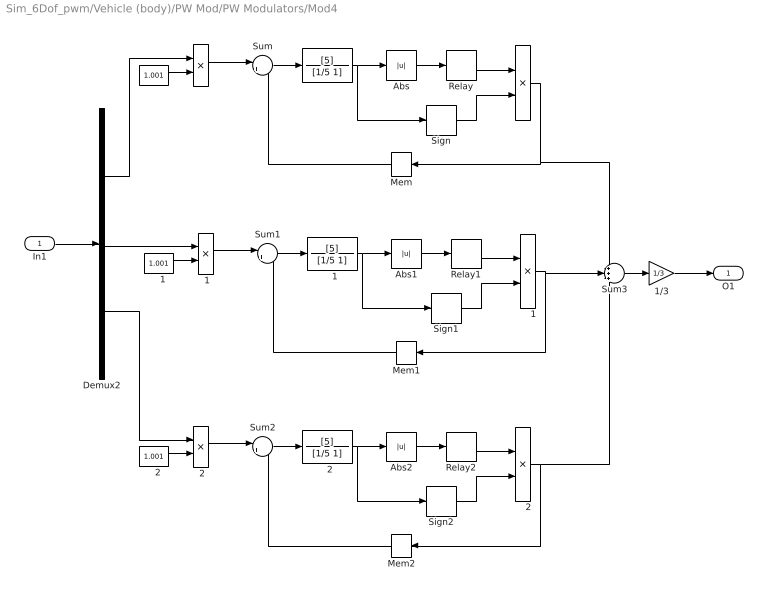
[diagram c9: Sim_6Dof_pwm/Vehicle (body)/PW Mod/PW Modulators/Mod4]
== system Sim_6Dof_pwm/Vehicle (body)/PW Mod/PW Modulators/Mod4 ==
  In1 : Inport  OutDataType=sfix(16)  OutScaling=2^0
  " " : Product  OutDataType=sfix(16)  OutScaling=2^0
  "  " : TransferFcn  Numerator=[5]  Denominator=[1/5 1]
  "   " : Constant  Value=1.001  OutDataType=sfix(16)  OutScaling=2^0
  "    " : Product  OutDataType=sfix(16)  OutScaling=2^0
  "    1" : Product  OutDataType=sfix(16)  OutScaling=2^0
  "    2" : Product  OutDataType=sfix(16)  OutScaling=2^0
  "   1" : Constant  Value=1.001  OutDataType=sfix(16)  OutScaling=2^0
  "   2" : Constant  Value=1.001  OutDataType=sfix(16)  OutScaling=2^0
  "  1" : TransferFcn  Numerator=[5]  Denominator=[1/5 1]
  "  2" : TransferFcn  Numerator=[5]  Denominator=[1/5 1]
  " 1" : Product  OutDataType=sfix(16)  OutScaling=2^0
  " 2" : Product  OutDataType=sfix(16)  OutScaling=2^0
  1/3 : Gain  Gain=1/3  ParameterDataType=sfix(16)  ParameterScaling=2^0  OutDataType=sfix(16)  OutScaling=2^0
  Abs : Abs
  Abs1 : Abs
  Abs2 : Abs
  Demux2 : Demux  Outputs=3
  Mem : Memory
  Mem1 : Memory
  Mem2 : Memory
  Relay : Relay  OnSwitchValue=0.5  OffSwitchValue=0.5  OutDataType=sfix(16)  OutScaling=2^0
  Relay1 : Relay  OnSwitchValue=0.5  OffSwitchValue=0.5  OutDataType=sfix(16)  OutScaling=2^0
  Relay2 : Relay  OnSwitchValue=0.5  OffSwitchValue=0.5  OutDataType=sfix(16)  OutScaling=2^0
  Sign : Signum
  Sign1 : Signum
  Sign2 : Signum
  Sum : Sum  Inputs=|+-  OutDataType=sfix(16)  OutScaling=2^0
  Sum1 : Sum  Inputs=|+-  OutDataType=sfix(16)  OutScaling=2^0
  Sum2 : Sum  Inputs=|+-  OutDataType=sfix(16)  OutScaling=2^0
  Sum3 : Sum  Inputs=+++  OutDataType=sfix(16)  OutScaling=2^0
  O1 : Outport  OutDataType=sfix(16)  OutScaling=2^0
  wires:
  "    "/1 -> Mem/1, Sum3/1
  Mem/1 -> Sum/2
  Sign/1 -> "    "/2
  Relay/1 -> "    "/1
  Abs/1 -> Relay/1
  "  "/1 -> Sign/1, Abs/1
  Sum/1 -> "  "/1
  "   "/1 -> " "/2
  " "/1 -> Sum/1
  "    1"/1 -> Mem1/1, Sum3/2
  Mem1/1 -> Sum1/2
  Sign1/1 -> "    1"/2
  Relay1/1 -> "    1"/1
  Abs1/1 -> Relay1/1
  "  1"/1 -> Sign1/1, Abs1/1
  Sum1/1 -> "  1"/1
  "   1"/1 -> " 1"/2
  " 1"/1 -> Sum1/1
  "    2"/1 -> Mem2/1, Sum3/3
  Mem2/1 -> Sum2/2
  Sign2/1 -> "    2"/2
  Relay2/1 -> "    2"/1
  Abs2/1 -> Relay2/1
  "  2"/1 -> Sign2/1, Abs2/1
  Sum2/1 -> "  2"/1
  "   2"/1 -> " 2"/2
  " 2"/1 -> Sum2/1
  Demux2/2 -> " 1"/1
  Demux2/1 -> " "/1
  Demux2/3 -> " 2"/1
  In1/1 -> Demux2/1
  Sum3/1 -> 1/3/1
  1/3/1 -> O1/1

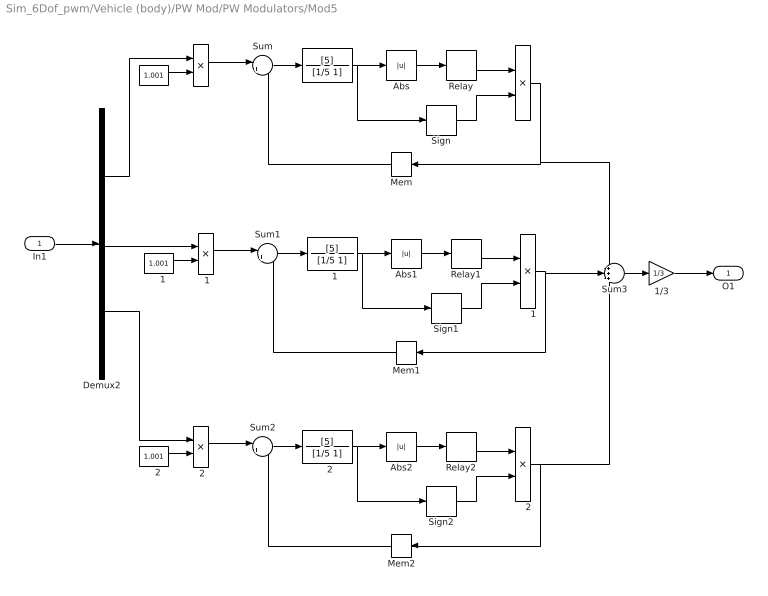
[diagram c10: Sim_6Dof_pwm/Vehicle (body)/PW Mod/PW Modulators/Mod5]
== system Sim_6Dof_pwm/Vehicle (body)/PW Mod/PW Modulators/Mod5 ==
  In1 : Inport  OutDataType=sfix(16)  OutScaling=2^0
  " " : Product  OutDataType=sfix(16)  OutScaling=2^0
  "  " : TransferFcn  Numerator=[5]  Denominator=[1/5 1]
  "   " : Constant  Value=1.001  OutDataType=sfix(16)  OutScaling=2^0
  "    " : Product  OutDataType=sfix(16)  OutScaling=2^0
  "    1" : Product  OutDataType=sfix(16)  OutScaling=2^0
  "    2" : Product  OutDataType=sfix(16)  OutScaling=2^0
  "   1" : Constant  Value=1.001  OutDataType=sfix(16)  OutScaling=2^0
  "   2" : Constant  Value=1.001  OutDataType=sfix(16)  OutScaling=2^0
  "  1" : TransferFcn  Numerator=[5]  Denominator=[1/5 1]
  "  2" : TransferFcn  Numerator=[5]  Denominator=[1/5 1]
  " 1" : Product  OutDataType=sfix(16)  OutScaling=2^0
  " 2" : Product  OutDataType=sfix(16)  OutScaling=2^0
  1/3 : Gain  Gain=1/3  ParameterDataType=sfix(16)  ParameterScaling=2^0  OutDataType=sfix(16)  OutScaling=2^0
  Abs : Abs
  Abs1 : Abs
  Abs2 : Abs
  Demux2 : Demux  Outputs=3
  Mem : Memory
  Mem1 : Memory
  Mem2 : Memory
  Relay : Relay  OnSwitchValue=0.5  OffSwitchValue=0.5  OutDataType=sfix(16)  OutScaling=2^0
  Relay1 : Relay  OnSwitchValue=0.5  OffSwitchValue=0.5  OutDataType=sfix(16)  OutScaling=2^0
  Relay2 : Relay  OnSwitchValue=0.5  OffSwitchValue=0.5  OutDataType=sfix(16)  OutScaling=2^0
  Sign : Signum
  Sign1 : Signum
  Sign2 : Signum
  Sum : Sum  Inputs=|+-  OutDataType=sfix(16)  OutScaling=2^0
  Sum1 : Sum  Inputs=|+-  OutDataType=sfix(16)  OutScaling=2^0
  Sum2 : Sum  Inputs=|+-  OutDataType=sfix(16)  OutScaling=2^0
  Sum3 : Sum  Inputs=+++  OutDataType=sfix(16)  OutScaling=2^0
  O1 : Outport  OutDataType=sfix(16)  OutScaling=2^0
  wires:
  "    "/1 -> Mem/1, Sum3/1
  Mem/1 -> Sum/2
  Sign/1 -> "    "/2
  Relay/1 -> "    "/1
  Abs/1 -> Relay/1
  "  "/1 -> Sign/1, Abs/1
  Sum/1 -> "  "/1
  "   "/1 -> " "/2
  " "/1 -> Sum/1
  "    1"/1 -> Mem1/1, Sum3/2
  Mem1/1 -> Sum1/2
  Sign1/1 -> "    1"/2
  Relay1/1 -> "    1"/1
  Abs1/1 -> Relay1/1
  "  1"/1 -> Sign1/1, Abs1/1
  Sum1/1 -> "  1"/1
  "   1"/1 -> " 1"/2
  " 1"/1 -> Sum1/1
  "    2"/1 -> Mem2/1, Sum3/3
  Mem2/1 -> Sum2/2
  Sign2/1 -> "    2"/2
  Relay2/1 -> "    2"/1
  Abs2/1 -> Relay2/1
  "  2"/1 -> Sign2/1, Abs2/1
  Sum2/1 -> "  2"/1
  "   2"/1 -> " 2"/2
  " 2"/1 -> Sum2/1
  Demux2/2 -> " 1"/1
  Demux2/1 -> " "/1
  Demux2/3 -> " 2"/1
  In1/1 -> Demux2/1
  Sum3/1 -> 1/3/1
  1/3/1 -> O1/1

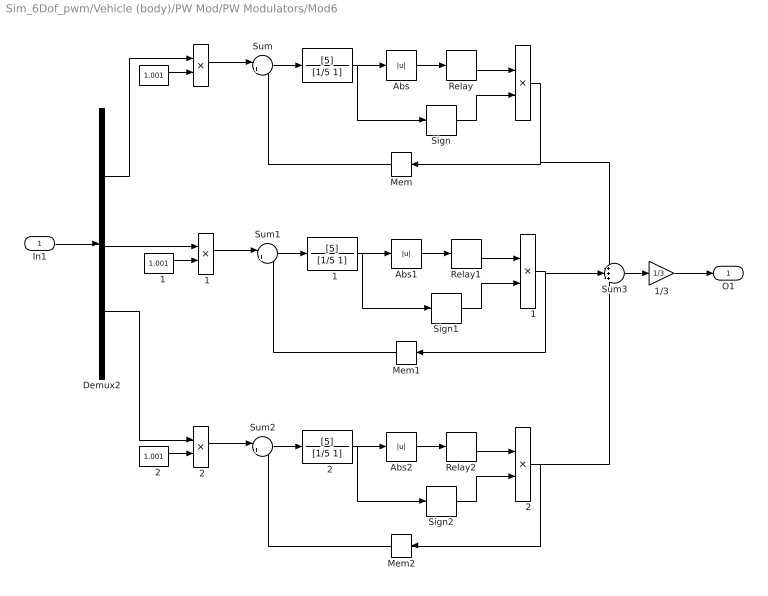
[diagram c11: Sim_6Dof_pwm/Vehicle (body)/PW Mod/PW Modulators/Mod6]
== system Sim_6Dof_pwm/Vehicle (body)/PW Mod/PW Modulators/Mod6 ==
  In1 : Inport  OutDataType=sfix(16)  OutScaling=2^0
  " " : Product  OutDataType=sfix(16)  OutScaling=2^0
  "  " : TransferFcn  Numerator=[5]  Denominator=[1/5 1]
  "   " : Constant  Value=1.001  OutDataType=sfix(16)  OutScaling=2^0
  "    " : Product  OutDataType=sfix(16)  OutScaling=2^0
  "    1" : Product  OutDataType=sfix(16)  OutScaling=2^0
  "    2" : Product  OutDataType=sfix(16)  OutScaling=2^0
  "   1" : Constant  Value=1.001  OutDataType=sfix(16)  OutScaling=2^0
  "   2" : Constant  Value=1.001  OutDataType=sfix(16)  OutScaling=2^0
  "  1" : TransferFcn  Numerator=[5]  Denominator=[1/5 1]
  "  2" : TransferFcn  Numerator=[5]  Denominator=[1/5 1]
  " 1" : Product  OutDataType=sfix(16)  OutScaling=2^0
  " 2" : Product  OutDataType=sfix(16)  OutScaling=2^0
  1/3 : Gain  Gain=1/3  ParameterDataType=sfix(16)  ParameterScaling=2^0  OutDataType=sfix(16)  OutScaling=2^0
  Abs : Abs
  Abs1 : Abs
  Abs2 : Abs
  Demux2 : Demux  Outputs=3
  Mem : Memory
  Mem1 : Memory
  Mem2 : Memory
  Relay : Relay  OnSwitchValue=0.5  OffSwitchValue=0.5  OutDataType=sfix(16)  OutScaling=2^0
  Relay1 : Relay  OnSwitchValue=0.5  OffSwitchValue=0.5  OutDataType=sfix(16)  OutScaling=2^0
  Relay2 : Relay  OnSwitchValue=0.5  OffSwitchValue=0.5  OutDataType=sfix(16)  OutScaling=2^0
  Sign : Signum
  Sign1 : Signum
  Sign2 : Signum
  Sum : Sum  Inputs=|+-  OutDataType=sfix(16)  OutScaling=2^0
  Sum1 : Sum  Inputs=|+-  OutDataType=sfix(16)  OutScaling=2^0
  Sum2 : Sum  Inputs=|+-  OutDataType=sfix(16)  OutScaling=2^0
  Sum3 : Sum  Inputs=+++  OutDataType=sfix(16)  OutScaling=2^0
  O1 : Outport  OutDataType=sfix(16)  OutScaling=2^0
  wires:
  "    "/1 -> Mem/1, Sum3/1
  Mem/1 -> Sum/2
  Sign/1 -> "    "/2
  Relay/1 -> "    "/1
  Abs/1 -> Relay/1
  "  "/1 -> Sign/1, Abs/1
  Sum/1 -> "  "/1
  "   "/1 -> " "/2
  " "/1 -> Sum/1
  "    1"/1 -> Mem1/1, Sum3/2
  Mem1/1 -> Sum1/2
  Sign1/1 -> "    1"/2
  Relay1/1 -> "    1"/1
  Abs1/1 -> Relay1/1
  "  1"/1 -> Sign1/1, Abs1/1
  Sum1/1 -> "  1"/1
  "   1"/1 -> " 1"/2
  " 1"/1 -> Sum1/1
  "    2"/1 -> Mem2/1, Sum3/3
  Mem2/1 -> Sum2/2
  Sign2/1 -> "    2"/2
  Relay2/1 -> "    2"/1
  Abs2/1 -> Relay2/1
  "  2"/1 -> Sign2/1, Abs2/1
  Sum2/1 -> "  2"/1
  "   2"/1 -> " 2"/2
  " 2"/1 -> Sum2/1
  Demux2/2 -> " 1"/1
  Demux2/1 -> " "/1
  Demux2/3 -> " 2"/1
  In1/1 -> Demux2/1
  Sum3/1 -> 1/3/1
  1/3/1 -> O1/1

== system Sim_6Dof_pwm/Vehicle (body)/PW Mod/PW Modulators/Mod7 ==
  In1 : Inport  OutDataType=sfix(16)  OutScaling=2^0
  " " : Product  OutDataType=sfix(16)  OutScaling=2^0
  "  " : TransferFcn  Numerator=[5]  Denominator=[1/5 1]
  "   " : Constant  Value=1.001  OutDataType=sfix(16)  OutScaling=2^0
  "    " : Product  OutDataType=sfix(16)  OutScaling=2^0
  "    1" : Product  OutDataType=sfix(16)  OutScaling=2^0
  "   1" : Constant  Value=1.001  OutDataType=sfix(16)  OutScaling=2^0
  "  1" : TransferFcn  Numerator=[5]  Denominator=[1/5 1]
  " 1" : Product  OutDataType=sfix(16)  OutScaling=2^0
  0.5 : Gain  Gain=0.5  ParameterDataType=sfix(16)  ParameterScaling=2^0  OutDataType=sfix(16)  OutScaling=2^0
  Abs : Abs
  Abs1 : Abs
  Demux2 : Demux  Outputs=2
  Mem : Memory
  Mem1 : Memory
  Relay : Relay  OnSwitchValue=0.5  OffSwitchValue=0.5  OutDataType=sfix(16)  OutScaling=2^0
  Relay1 : Relay  OnSwitchValue=0.5  OffSwitchValue=0.5  OutDataType=sfix(16)  OutScaling=2^0
  Sign : Signum
  Sign1 : Signum
  Sum : Sum  Inputs=|+-  OutDataType=sfix(16)  OutScaling=2^0
  Sum1 : Sum  Inputs=|+-  OutDataType=sfix(16)  OutScaling=2^0
  Sum3 : Sum  Inputs=++|  OutDataType=sfix(16)  OutScaling=2^0
  O1 : Outport  OutDataType=sfix(16)  OutScaling=2^0
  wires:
  "    "/1 -> Mem/1, Sum3/1
  Mem/1 -> Sum/2
  Sign/1 -> "    "/2
  Relay/1 -> "    "/1
  Abs/1 -> Relay/1
  "  "/1 -> Sign/1, Abs/1
  Sum/1 -> "  "/1
  "   "/1 -> " "/2
  " "/1 -> Sum/1
  "    1"/1 -> Mem1/1, Sum3/2
  Mem1/1 -> Sum1/2
  Sign1/1 -> "    1"/2
  Relay1/1 -> "    1"/1
  Abs1/1 -> Relay1/1
  "  1"/1 -> Sign1/1, Abs1/1
  Sum1/1 -> "  1"/1
  "   1"/1 -> " 1"/2
  " 1"/1 -> Sum1/1
  Demux2/2 -> " 1"/1
  Demux2/1 -> " "/1
  In1/1 -> Demux2/1
  Sum3/1 -> 0.5/1
  0.5/1 -> O1/1

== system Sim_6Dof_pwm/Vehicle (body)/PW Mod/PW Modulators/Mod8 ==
  In1 : Inport  OutDataType=sfix(16)  OutScaling=2^0
  " " : Product  OutDataType=sfix(16)  OutScaling=2^0
  "  " : TransferFcn  Numerator=[5]  Denominator=[1/5 1]
  "   " : Constant  Value=1.001  OutDataType=sfix(16)  OutScaling=2^0
  "    " : Product  OutDataType=sfix(16)  OutScaling=2^0
  "    1" : Product  OutDataType=sfix(16)  OutScaling=2^0
  "   1" : Constant  Value=1.001  OutDataType=sfix(16)  OutScaling=2^0
  "  1" : TransferFcn  Numerator=[5]  Denominator=[1/5 1]
  " 1" : Product  OutDataType=sfix(16)  OutScaling=2^0
  0.5 : Gain  Gain=0.5  ParameterDataType=sfix(16)  ParameterScaling=2^0  OutDataType=sfix(16)  OutScaling=2^0
  Abs : Abs
  Abs1 : Abs
  Demux2 : Demux  Outputs=2
  Mem : Memory
  Mem1 : Memory
  Relay : Relay  OnSwitchValue=0.5  OffSwitchValue=0.5  OutDataType=sfix(16)  OutScaling=2^0
  Relay1 : Relay  OnSwitchValue=0.5  OffSwitchValue=0.5  OutDataType=sfix(16)  OutScaling=2^0
  Sign : Signum
  Sign1 : Signum
  Sum : Sum  Inputs=|+-  OutDataType=sfix(16)  OutScaling=2^0
  Sum1 : Sum  Inputs=|+-  OutDataType=sfix(16)  OutScaling=2^0
  Sum3 : Sum  Inputs=++|  OutDataType=sfix(16)  OutScaling=2^0
  O1 : Outport  OutDataType=sfix(16)  OutScaling=2^0
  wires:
  "    "/1 -> Mem/1, Sum3/1
  Mem/1 -> Sum/2
  Sign/1 -> "    "/2
  Relay/1 -> "    "/1
  Abs/1 -> Relay/1
  "  "/1 -> Sign/1, Abs/1
  Sum/1 -> "  "/1
  "   "/1 -> " "/2
  " "/1 -> Sum/1
  "    1"/1 -> Mem1/1, Sum3/2
  Mem1/1 -> Sum1/2
  Sign1/1 -> "    1"/2
  Relay1/1 -> "    1"/1
  Abs1/1 -> Relay1/1
  "  1"/1 -> Sign1/1, Abs1/1
  Sum1/1 -> "  1"/1
  "   1"/1 -> " 1"/2
  " 1"/1 -> Sum1/1
  Demux2/2 -> " 1"/1
  Demux2/1 -> " "/1
  In1/1 -> Demux2/1
  Sum3/1 -> 0.5/1
  0.5/1 -> O1/1

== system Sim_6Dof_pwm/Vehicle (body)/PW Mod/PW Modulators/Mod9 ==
  In1 : Inport  OutDataType=sfix(16)  OutScaling=2^0
  " " : Product  OutDataType=sfix(16)  OutScaling=2^0
  "  " : TransferFcn  Numerator=[5]  Denominator=[1/5 1]
  "   " : Constant  Value=1.001  OutDataType=sfix(16)  OutScaling=2^0
  "    " : Product  OutDataType=sfix(16)  OutScaling=2^0
  "    1" : Product  OutDataType=sfix(16)  OutScaling=2^0
  "   1" : Constant  Value=1.001  OutDataType=sfix(16)  OutScaling=2^0
  "  1" : TransferFcn  Numerator=[5]  Denominator=[1/5 1]
  " 1" : Product  OutDataType=sfix(16)  OutScaling=2^0
  0.5 : Gain  Gain=0.5  ParameterDataType=sfix(16)  ParameterScaling=2^0  OutDataType=sfix(16)  OutScaling=2^0
  Abs : Abs
  Abs1 : Abs
  Demux2 : Demux  Outputs=2
  Mem : Memory
  Mem1 : Memory
  Relay : Relay  OnSwitchValue=0.5  OffSwitchValue=0.5  OutDataType=sfix(16)  OutScaling=2^0
  Relay1 : Relay  OnSwitchValue=0.5  OffSwitchValue=0.5  OutDataType=sfix(16)  OutScaling=2^0
  Sign : Signum
  Sign1 : Signum
  Sum : Sum  Inputs=|+-  OutDataType=sfix(16)  OutScaling=2^0
  Sum1 : Sum  Inputs=|+-  OutDataType=sfix(16)  OutScaling=2^0
  Sum3 : Sum  Inputs=++|  OutDataType=sfix(16)  OutScaling=2^0
  O1 : Outport  OutDataType=sfix(16)  OutScaling=2^0
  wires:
  "    "/1 -> Mem/1, Sum3/1
  Mem/1 -> Sum/2
  Sign/1 -> "    "/2
  Relay/1 -> "    "/1
  Abs/1 -> Relay/1
  "  "/1 -> Sign/1, Abs/1
  Sum/1 -> "  "/1
  "   "/1 -> " "/2
  " "/1 -> Sum/1
  "    1"/1 -> Mem1/1, Sum3/2
  Mem1/1 -> Sum1/2
  Sign1/1 -> "    1"/2
  Relay1/1 -> "    1"/1
  Abs1/1 -> Relay1/1
  "  1"/1 -> Sign1/1, Abs1/1
  Sum1/1 -> "  1"/1
  "   1"/1 -> " 1"/2
  " 1"/1 -> Sum1/1
  Demux2/2 -> " 1"/1
  Demux2/1 -> " "/1
  In1/1 -> Demux2/1
  Sum3/1 -> 0.5/1
  0.5/1 -> O1/1
